FUNCTION "FC_GRP_82_R14" : VOID
TITLE =GROUP =82_R14
VERSION : 0.1


VAR_TEMP
  CL : "UDT_CABINET";	//CABINET LOCAL
  CR : "UDT_CABINET";	//CABINET REMOTE
  RelError : BOOL ;	//ERROR RELEASE
  RelErrorCL : BOOL ;	//ERROR RELEASE FROM CABINET LOCAL
  RelErrorCR : BOOL ;	//ERROR RELEASE FROM CABINET REMOTE
  RelControl : BOOL ;	//CONTROL RELEASE
  RelControlCL : BOOL ;	//CONTROL RELEASE FROM CABINET LOCAL
  RelControlCR : BOOL ;	//CONTROL RELEASE FROM CABINET REMOTE
  ErrorConfirm : BOOL ;	//ERROR CONFIRM
  AutoOn : BOOL ;	//AUTOMATIC ON
  AutoOff : BOOL ;	//AUTOMATIC OFF
  RelAuto : BOOL ;	//AUTOMATIC RELEASE
  TempSetpoint : WORD ;
  LAMP_ON : BOOL ;
END_VAR
BEGIN
NETWORK
TITLE =GLOBAL SIGNALS
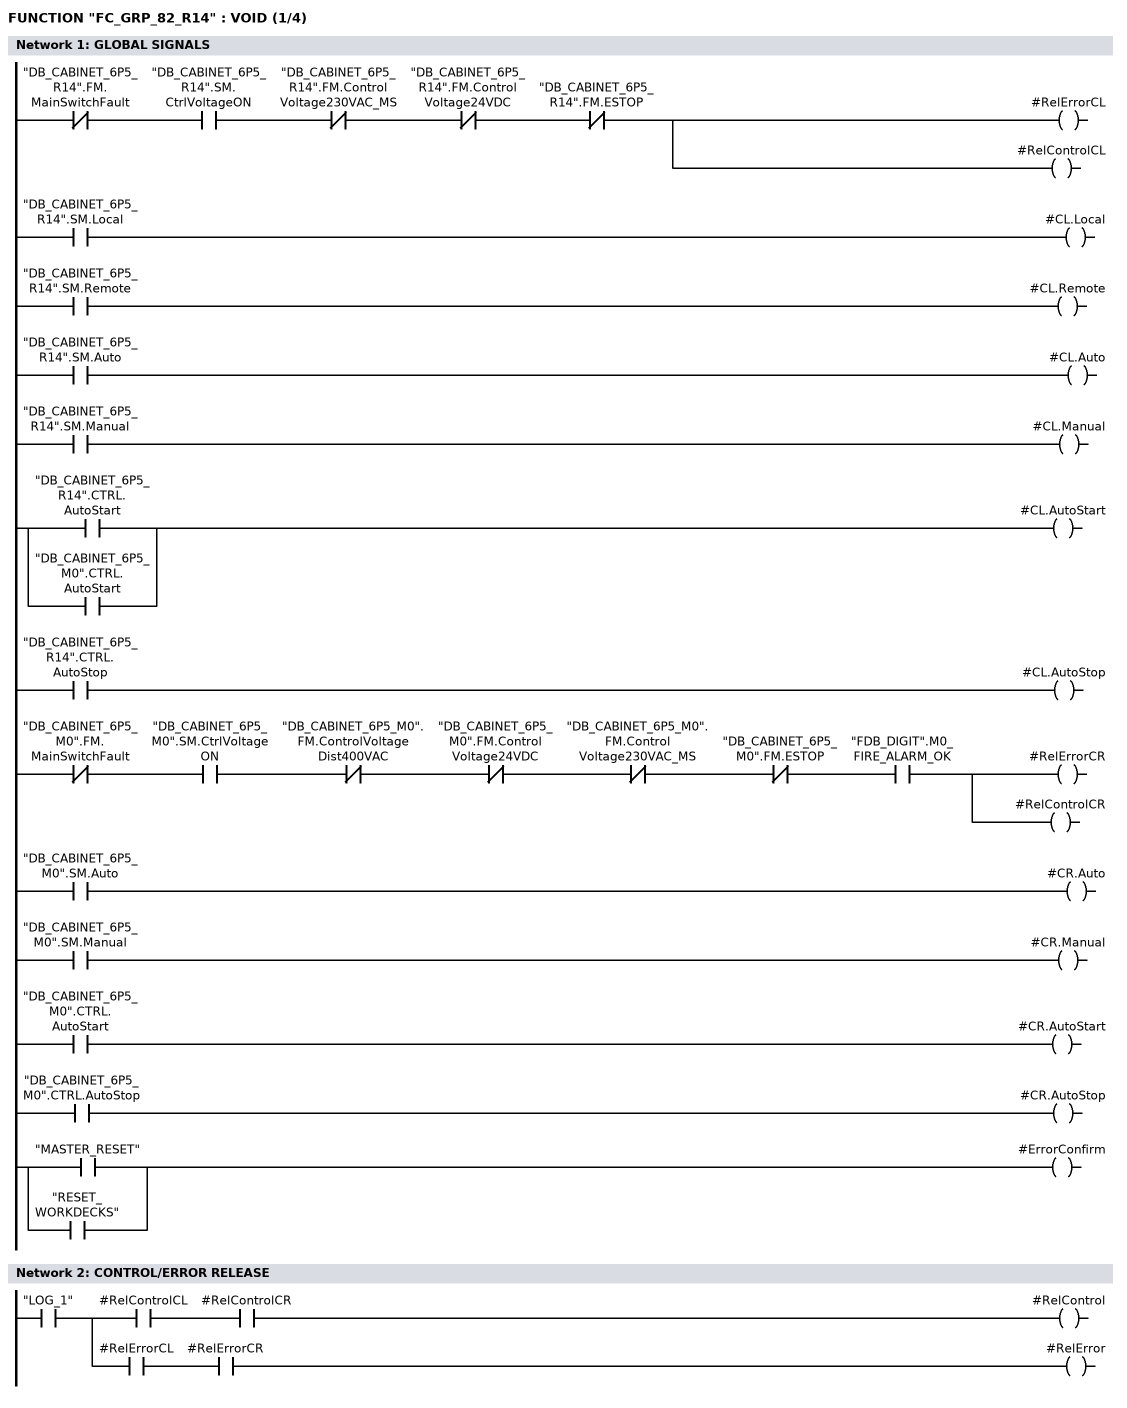
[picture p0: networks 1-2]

      UN    "DB_CABINET_6P5_R14".FM.MainSwitchFault;
      U     "DB_CABINET_6P5_R14".SM.CtrlVoltageON;
      UN    "DB_CABINET_6P5_R14".FM.ControlVoltage230VAC_MS;
      UN    "DB_CABINET_6P5_R14".FM.ControlVoltage24VDC;
      UN    "DB_CABINET_6P5_R14".FM.ESTOP;
      =     #RelErrorCL;
      =     #RelControlCL;

      U     "DB_CABINET_6P5_R14".SM.Local;
      =     #CL.Local;
      U     "DB_CABINET_6P5_R14".SM.Remote;
      =     #CL.Remote;
      U     "DB_CABINET_6P5_R14".SM.Auto;
      =     #CL.Auto;
      U     "DB_CABINET_6P5_R14".SM.Manual;
      =     #CL.Manual;
      U     "DB_CABINET_6P5_R14".CTRL.AutoStart;
      O     "DB_CABINET_6P5_M0".CTRL.AutoStart;
      =     #CL.AutoStart;
      U     "DB_CABINET_6P5_R14".CTRL.AutoStop;
      =     #CL.AutoStop;


      UN    "DB_CABINET_6P5_M0".FM.MainSwitchFault;
      U     "DB_CABINET_6P5_M0".SM.CtrlVoltageON;
      UN    "DB_CABINET_6P5_M0".FM.ControlVoltageDist400VAC;
      UN    "DB_CABINET_6P5_M0".FM.ControlVoltage24VDC;
      UN    "DB_CABINET_6P5_M0".FM.ControlVoltage230VAC_MS;
      UN    "DB_CABINET_6P5_M0".FM.ESTOP;
      U     "FDB_DIGIT".M0_FIRE_ALARM_OK;
      =     #RelErrorCR;
      =     #RelControlCR;

      U     "DB_CABINET_6P5_M0".SM.Auto;
      =     #CR.Auto;
      U     "DB_CABINET_6P5_M0".SM.Manual;
      =     #CR.Manual;
      U     "DB_CABINET_6P5_M0".CTRL.AutoStart;
      =     #CR.AutoStart;
      U     "DB_CABINET_6P5_M0".CTRL.AutoStop;
      =     #CR.AutoStop;


      U     "MASTER_RESET";
      O     "RESET_WORKDECKS";
      =     #ErrorConfirm;

NETWORK
TITLE =CONTROL/ERROR RELEASE

      U     "LOG_1";
      =     L      9.0;
      U     L      9.0;
      U     #RelControlCL;
      U     #RelControlCR;
      =     #RelControl;
      U     L      9.0;
      U     #RelErrorCL;
      U     #RelErrorCR;
      =     #RelError;
NETWORK
TITLE =SUPPLY AIR FAN =82FAN02, CONTROL SIGNALS
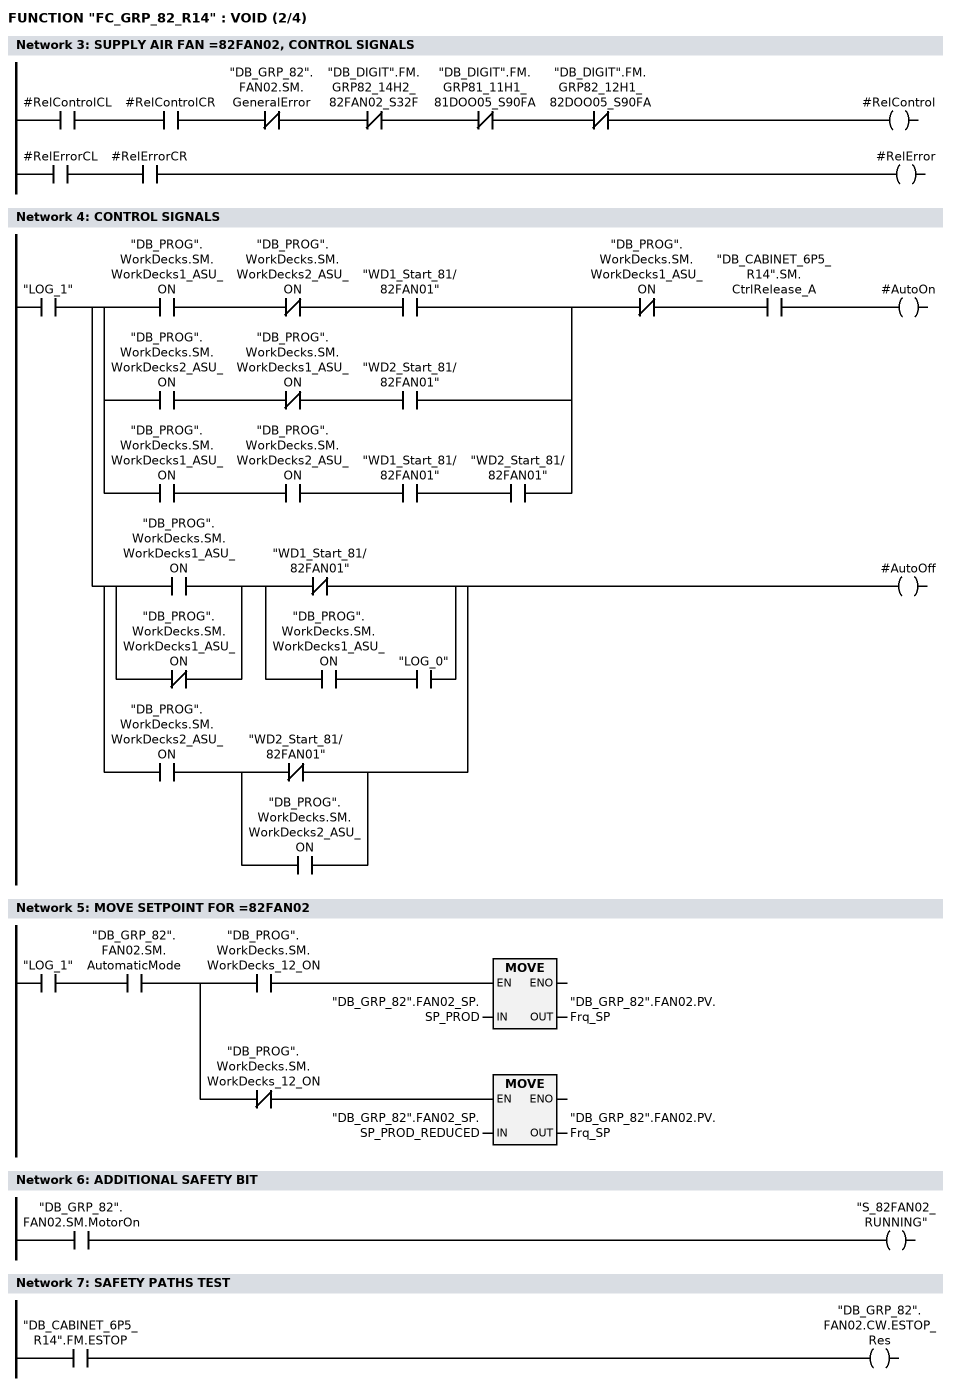
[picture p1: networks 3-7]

      U     #RelControlCL;
      U     #RelControlCR;
      UN    "DB_GRP_82".FAN02.SM.GeneralError;
      UN    "DB_DIGIT".FM.GRP82_14H2_82FAN02_S32F;
//   AN    "6P5_82FAN02+14H2-A85:31"
      UN    "DB_DIGIT".FM.GRP81_11H1_81DOO05_S90FA;
      UN    "DB_DIGIT".FM.GRP82_12H1_82DOO05_S90FA;
      =     #RelControl;

      U     #RelErrorCL;
      U     #RelErrorCR;
      =     #RelError;


NETWORK
TITLE =CONTROL SIGNALS

      U     "LOG_1";
      =     L      9.0;
      U     L      9.0;
      U(    ;
      U     "DB_PROG".WorkDecks.SM.WorkDecks1_ASU_ON;
      UN    "DB_PROG".WorkDecks.SM.WorkDecks2_ASU_ON;
      U     "WD1_Start_81/82FAN01";
      O     ;
      U     "DB_PROG".WorkDecks.SM.WorkDecks2_ASU_ON;
      UN    "DB_PROG".WorkDecks.SM.WorkDecks1_ASU_ON;
      U     "WD2_Start_81/82FAN01";
      O     ;
      U     "DB_PROG".WorkDecks.SM.WorkDecks1_ASU_ON;
      U     "DB_PROG".WorkDecks.SM.WorkDecks2_ASU_ON;
      U     "WD1_Start_81/82FAN01";
      U     "WD2_Start_81/82FAN01";
      )     ;
      UN    "DB_PROG".WorkDecks.SM.WorkDecks1_ASU_ON;
      U     "DB_CABINET_6P5_R14".SM.CtrlRelease_A;
      =     #AutoOn;
      U     L      9.0;
      U(    ;
      U(    ;
      O     "DB_PROG".WorkDecks.SM.WorkDecks1_ASU_ON;
      ON    "DB_PROG".WorkDecks.SM.WorkDecks1_ASU_ON;
      )     ;
      U(    ;
      ON    "WD1_Start_81/82FAN01";
      O     ;
      U     "DB_PROG".WorkDecks.SM.WorkDecks1_ASU_ON;
      U     "LOG_0";
      )     ;
      O     ;
      U     "DB_PROG".WorkDecks.SM.WorkDecks2_ASU_ON;
      U(    ;
      ON    "WD2_Start_81/82FAN01";
      O     "DB_PROG".WorkDecks.SM.WorkDecks2_ASU_ON;
      )     ;
      )     ;
      =     #AutoOff;
NETWORK
TITLE =MOVE SETPOINT FOR =82FAN02

      U     "LOG_1";
      U     "DB_GRP_82".FAN02.SM.AutomaticMode;
      =     L      9.0;
      U     L      9.0;
      U     "DB_PROG".WorkDecks.SM.WorkDecks_12_ON;
      SPBNB _001;
      L     "DB_GRP_82".FAN02_SP.SP_PROD;
      T     "DB_GRP_82".FAN02.PV.Frq_SP;
_001: NOP   0;
      U     L      9.0;
      UN    "DB_PROG".WorkDecks.SM.WorkDecks_12_ON;
      SPBNB _002;
      L     "DB_GRP_82".FAN02_SP.SP_PROD_REDUCED;
      T     "DB_GRP_82".FAN02.PV.Frq_SP;
_002: NOP   0;
NETWORK
TITLE =ADDITIONAL SAFETY BIT

      U     "DB_GRP_82".FAN02.SM.MotorOn;
      =     "S_82FAN02_RUNNING";
NETWORK
TITLE =SAFETY PATHS TEST

      U     "DB_CABINET_6P5_R14".FM.ESTOP;
      =     "DB_GRP_82".FAN02.CW.ESTOP_Res;
NETWORK
TITLE =COAST DOWN ENABLED 82FAN02
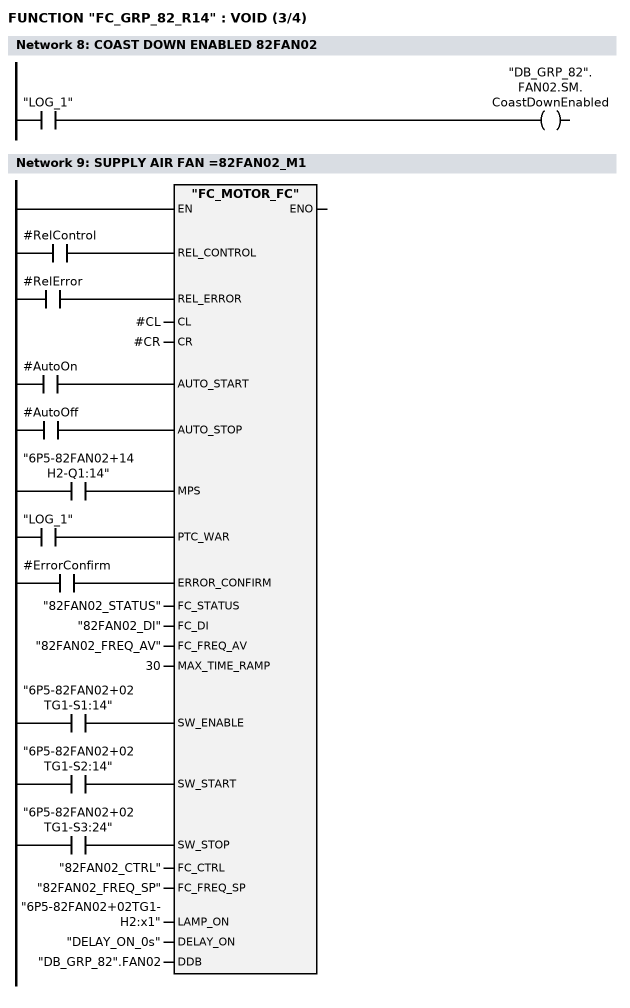
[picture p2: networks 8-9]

      U     "LOG_1";
      =     "DB_GRP_82".FAN02.SM.CoastDownEnabled;
NETWORK
TITLE =SUPPLY AIR FAN =82FAN02_M1

      U     #RelControl;
      =     L      9.0;
      BLD   103;
      U     #RelError;
      =     L      9.1;
      BLD   103;
      U     #AutoOn;
      =     L      9.2;
      BLD   103;
      U     #AutoOff;
      =     L      9.3;
      BLD   103;
      U     "6P5-82FAN02+14H2-Q1:14";
      =     L      9.4;
      BLD   103;
      U     "LOG_1";
      =     L      9.5;
      BLD   103;
      U     #ErrorConfirm;
      =     L      9.6;
      BLD   103;
      U     "6P5-82FAN02+02TG1-S1:14";
      =     L      9.7;
      BLD   103;
      U     "6P5-82FAN02+02TG1-S2:14";
      =     L     10.0;
      BLD   103;
      U     "6P5-82FAN02+02TG1-S3:24";
      =     L     10.1;
      BLD   103;
      CALL "FC_MOTOR_FC" (
           REL_CONTROL              := L      9.0,
           REL_ERROR                := L      9.1,
           CL                       := #CL,
           CR                       := #CR,
           AUTO_START               := L      9.2,
           AUTO_STOP                := L      9.3,
           MPS                      := L      9.4,
           PTC_WAR                  := L      9.5,
           ERROR_CONFIRM            := L      9.6,
           FC_STATUS                := "82FAN02_STATUS",
           FC_DI                    := "82FAN02_DI",
           FC_FREQ_AV               := "82FAN02_FREQ_AV",
           MAX_TIME_RAMP            := 30,
           SW_ENABLE                := L      9.7,
           SW_START                 := L     10.0,
           SW_STOP                  := L     10.1,
           FC_CTRL                  := "82FAN02_CTRL",
           FC_FREQ_SP               := "82FAN02_FREQ_SP",
           LAMP_ON                  := "6P5-82FAN02+02TG1-H2:x1",
           DELAY_ON                 := "DELAY_ON_0s",
           DDB                      := "DB_GRP_82".FAN02);
      NOP   0;
NETWORK
TITLE =PRESSURE SENSOR, =82FAN02_S32F
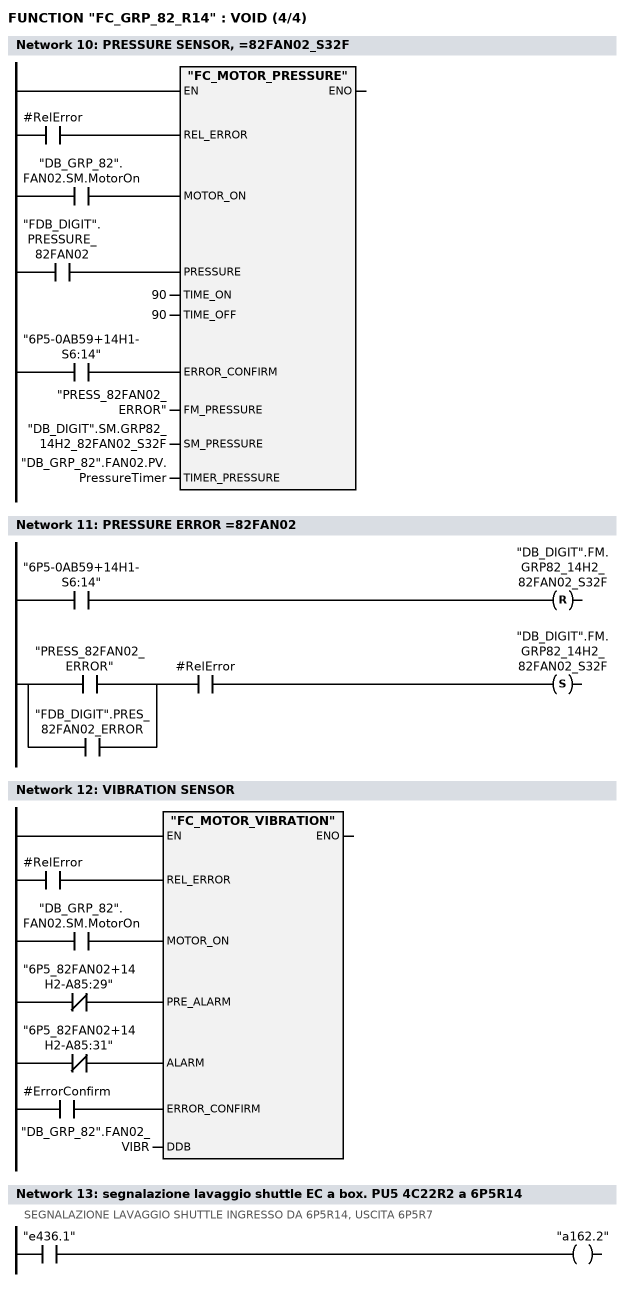
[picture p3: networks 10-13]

      U     #RelError;
      =     L      9.0;
      BLD   103;
      U     "DB_GRP_82".FAN02.SM.MotorOn;
      =     L      9.1;
      BLD   103;
      U     "FDB_DIGIT".PRESSURE_82FAN02;
      =     L      9.2;
      BLD   103;
      U     "6P5-0AB59+14H1-S6:14";
      =     L      9.3;
      BLD   103;
      CALL "FC_MOTOR_PRESSURE" (
           REL_ERROR                := L      9.0,
           MOTOR_ON                 := L      9.1,
           PRESSURE                 := L      9.2,
           TIME_ON                  := 90,
           TIME_OFF                 := 90,
           ERROR_CONFIRM            := L      9.3,
           FM_PRESSURE              := "PRESS_82FAN02_ERROR",
           SM_PRESSURE              := "DB_DIGIT".SM.GRP82_14H2_82FAN02_S32F,
           TIMER_PRESSURE           := "DB_GRP_82".FAN02.PV.PressureTimer);
      NOP   0;
NETWORK
TITLE =PRESSURE ERROR =82FAN02

      U     "6P5-0AB59+14H1-S6:14";
      R     "DB_DIGIT".FM.GRP82_14H2_82FAN02_S32F;
      U(    ;
      O     "PRESS_82FAN02_ERROR";
      O     "FDB_DIGIT".PRES_82FAN02_ERROR;
      )     ;
      U     #RelError;
      S     "DB_DIGIT".FM.GRP82_14H2_82FAN02_S32F;
      NOP   0;
NETWORK
TITLE =VIBRATION SENSOR

      U     #RelError;
      =     L      9.0;
      BLD   103;
      U     "DB_GRP_82".FAN02.SM.MotorOn;
      =     L      9.1;
      BLD   103;
      UN    "6P5_82FAN02+14H2-A85:29";
      =     L      9.2;
      BLD   103;
      UN    "6P5_82FAN02+14H2-A85:31";
      =     L      9.3;
      BLD   103;
      U     #ErrorConfirm;
      =     L      9.4;
      BLD   103;
      CALL "FC_MOTOR_VIBRATION" (
           REL_ERROR                := L      9.0,
           MOTOR_ON                 := L      9.1,
           PRE_ALARM                := L      9.2,
           ALARM                    := L      9.3,
           ERROR_CONFIRM            := L      9.4,
           DDB                      := "DB_GRP_82".FAN02_VIBR);
      NOP   0;
NETWORK
TITLE =segnalazione lavaggio shuttle EC a box. PU5 4C22R2 a 6P5R14
//SEGNALAZIONE LAVAGGIO SHUTTLE INGRESSO DA 6P5R14, USCITA 6P5R7
      U     "e436.1";
      =     "a162.2";
NETWORK
TITLE =END

END_FUNCTION

